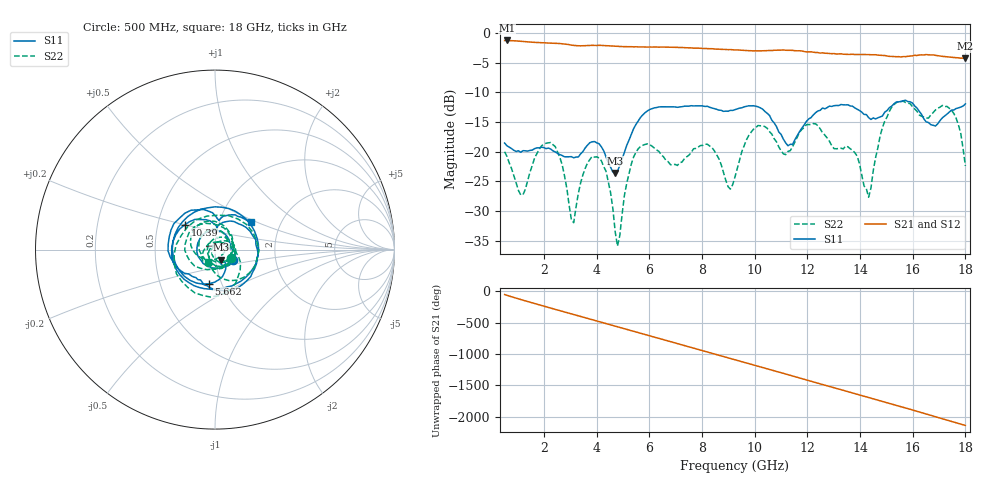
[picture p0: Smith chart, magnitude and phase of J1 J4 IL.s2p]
!Agilent Technologies,N5230A,MY45001360,A.07.50.67
!Agilent N5230A: A.07.50.67
!Date: Tuesday, April 16, 2024 17:37:33
!Correction: S11(Full 2 Port(1,2))
!S21(Full 2 Port(1,2))
!S12(Full 2 Port(1,2))
!S22(Full 2 Port(1,2))
!S2P File: Measurements: S11, S21, S12, S22:
# Hz S  dB  R 50
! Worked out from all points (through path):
!   201 points, 500 MHz to 18 GHz, reference 50 ohm
!   highest |S21| = -1.26 dB at 587.5 MHz (marker M1); lowest = -4.3 dB at 18 GHz (marker M2)
!   group delay of S21, straight-line fit = 329 ps
!   lowest |S11| = -23.6 dB at 4.7 GHz (marker M3), VSWR 1.14, Z = 53.2 - j6.06 ohm
!   |S11| at or under -10 dB: start of sweep to end of sweep
!   |S22| runs from -35.9 to -11.5 dB; largest |S21 - S12| = 0.0082
!   S11 on the Smith chart (normalised r, x): 500 MHz: 1.22, -0.15; 5.662 GHz: 0.87, -0.34; 10.39 GHz: 0.69, +0.20; 18 GHz: 1.41, +0.46
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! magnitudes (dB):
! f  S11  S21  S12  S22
! 500 MHz  -18.6  -1.3  -1.3  -20.0
! 587.5 MHz  -19.0  -1.3  -1.3  -20.8
! 1.2 GHz  -19.8  -1.4  -1.4  -27.2
! 2.425 GHz  -20.1  -1.7  -1.7  -19.2
! 3.125 GHz  -21.0  -2.1  -2.1  -32.0
! 3.475 GHz  -20.0  -2.2  -2.1  -23.9
! 4.175 GHz  -19.2  -2.1  -2.1  -21.5
! 4.7 GHz  -23.6  -2.2  -2.2  -33.5
! 4.787 GHz  -23.3  -2.3  -2.3  -35.9
! 5.138 GHz  -19.0  -2.3  -2.3  -25.4
! 5.662 GHz  -14.2  -2.3  -2.3  -19.1
! 6.362 GHz  -12.5  -2.4  -2.4  -20.0
! 8.2 GHz  -12.4  -2.6  -2.7  -18.8
! 9.25 GHz  -12.9  -2.9  -2.9  -24.2
! 10.39 GHz  -13.2  -3.0  -3.0  -15.8
! 11.26 GHz  -19.0  -2.9  -2.9  -20.0
! 12.22 GHz  -13.8  -3.2  -3.2  -15.3
! 13.8 GHz  -12.6  -3.6  -3.6  -20.2
! 14.32 GHz  -14.3  -3.6  -3.6  -27.7
! 15.11 GHz  -12.6  -4.0  -3.9  -13.2
! 17.3 GHz  -13.7  -4.0  -4.0  -12.4
! 18 GHz  -11.9  -4.3  -4.3  -22.4
